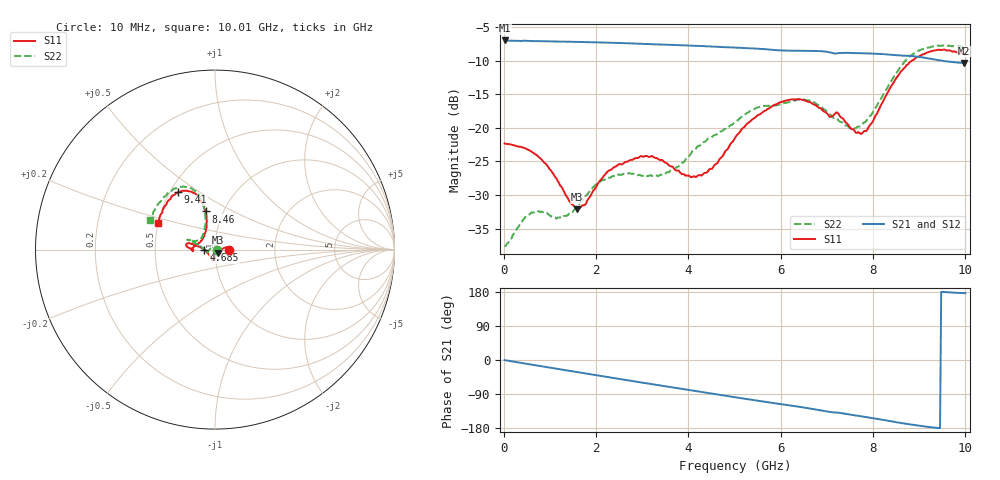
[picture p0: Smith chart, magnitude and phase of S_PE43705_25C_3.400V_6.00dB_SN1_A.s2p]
! Device ID: PE43705
! Serial: 1
! Insertion: A
! Impedance: 50 ohm
! Temp: 25C
! VDD: 3.400V
! Attenuation Step: 6.00dB
#  Hz  S  RI  R  50
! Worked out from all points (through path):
!   401 points, 10 MHz to 10.01 GHz, reference 50 ohm
!   highest |S21| = -7.00 dB at 10 MHz (marker M1); lowest = -10.3 dB at 9.985 GHz (marker M2)
!   group delay of S21, straight-line fit = 52.4 ps
!   lowest |S11| = -32.2 dB at 1.585 GHz (marker M3), VSWR 1.05, Z = 51.9 - j1.68 ohm
!   |S11| at or under -10 dB: start of sweep to 8.852 GHz
!   |S22| runs from -37.6 to -7.7 dB; largest |S21 - S12| = 0.004
!   S11 on the Smith chart (normalised r, x): 10 MHz: 1.17, -0.00; 4.685 GHz: 0.89, -0.00; 8.46 GHz: 0.83, +0.37; 9.41 GHz: 0.55, +0.41; 10.01 GHz: 0.50, +0.17
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1e7  0.0764 -0.000236  0.4468 -0.00217  0.4472 -0.00208  0.0132 0.000294
5.85e8  0.0655 0.0131  0.4325 -0.0918  0.4326 -0.0917  0.00829 0.0219
1.21e9  0.0374 0.000605  0.3992 -0.1814  0.3992 -0.1811  -0.0123 0.0176
1.585e9  0.0186 -0.0162  0.3698 -0.2303  0.3699 -0.2302  -0.025 0.00603
1.685e9  0.0145 -0.0219  0.3612 -0.2426  0.3613 -0.2424  -0.0287 0.00234
2.06e9  0.00045 -0.0395  0.3247 -0.2851  0.3246 -0.2848  -0.0381 -0.00957
2.435e9  -0.00489 -0.0515  0.2828 -0.3217  0.2829 -0.3217  -0.0411 -0.0155
3.36e9  -0.0139 -0.0565  0.1654 -0.3829  0.1659 -0.3826  -0.0422 -0.0121
4.11e9  -0.0324 -0.0288  0.0634 -0.4036  0.0642 -0.4034  -0.0674 0.00613
4.685e9  -0.0589 -0.00169  -0.015 -0.3991  -0.0141 -0.3993  -0.0907 0.0228
5.01e9  -0.0827 0.0149  -0.0566 -0.3912  -0.0561 -0.3914  -0.106 0.0324
5.46e9  -0.1172 0.0273  -0.1124 -0.3726  -0.1121 -0.3726  -0.1313 0.0489
5.935e9  -0.1472 0.036  -0.1614 -0.3414  -0.1603 -0.3421  -0.1377 0.0536
6.685e9  -0.1509 0.0126  -0.2351 -0.2901  -0.2351 -0.29  -0.146 0.0531
7.46e9  -0.1025 0.0277  -0.2892 -0.2163  -0.2886 -0.2168  -0.0861 0.0565
7.76e9  -0.0699 0.0573  -0.3071 -0.1853  -0.3062 -0.1864  -0.0675 0.0807
8.36e9  -0.0474 0.1874  -0.3312 -0.1154  -0.3304 -0.1165  -0.056 0.2048
8.46e9  -0.0521 0.2126  -0.3327 -0.1014  -0.3321 -0.1031  -0.0611 0.233
8.86e9  -0.1026 0.3006  -0.3372 -0.0544  -0.3346 -0.0559  -0.1187 0.3307
9.41e9  -0.2065 0.3191  -0.3198 -0.00343  -0.319 -0.00368  -0.2297 0.3384
9.985e9  -0.3122 0.1586  -0.3032 0.0186  -0.3039 0.0182  -0.3531 0.1768
1.001e10  -0.3191 0.1487  -0.3046 0.0192  -0.3054 0.0186  -0.3608 0.1655
